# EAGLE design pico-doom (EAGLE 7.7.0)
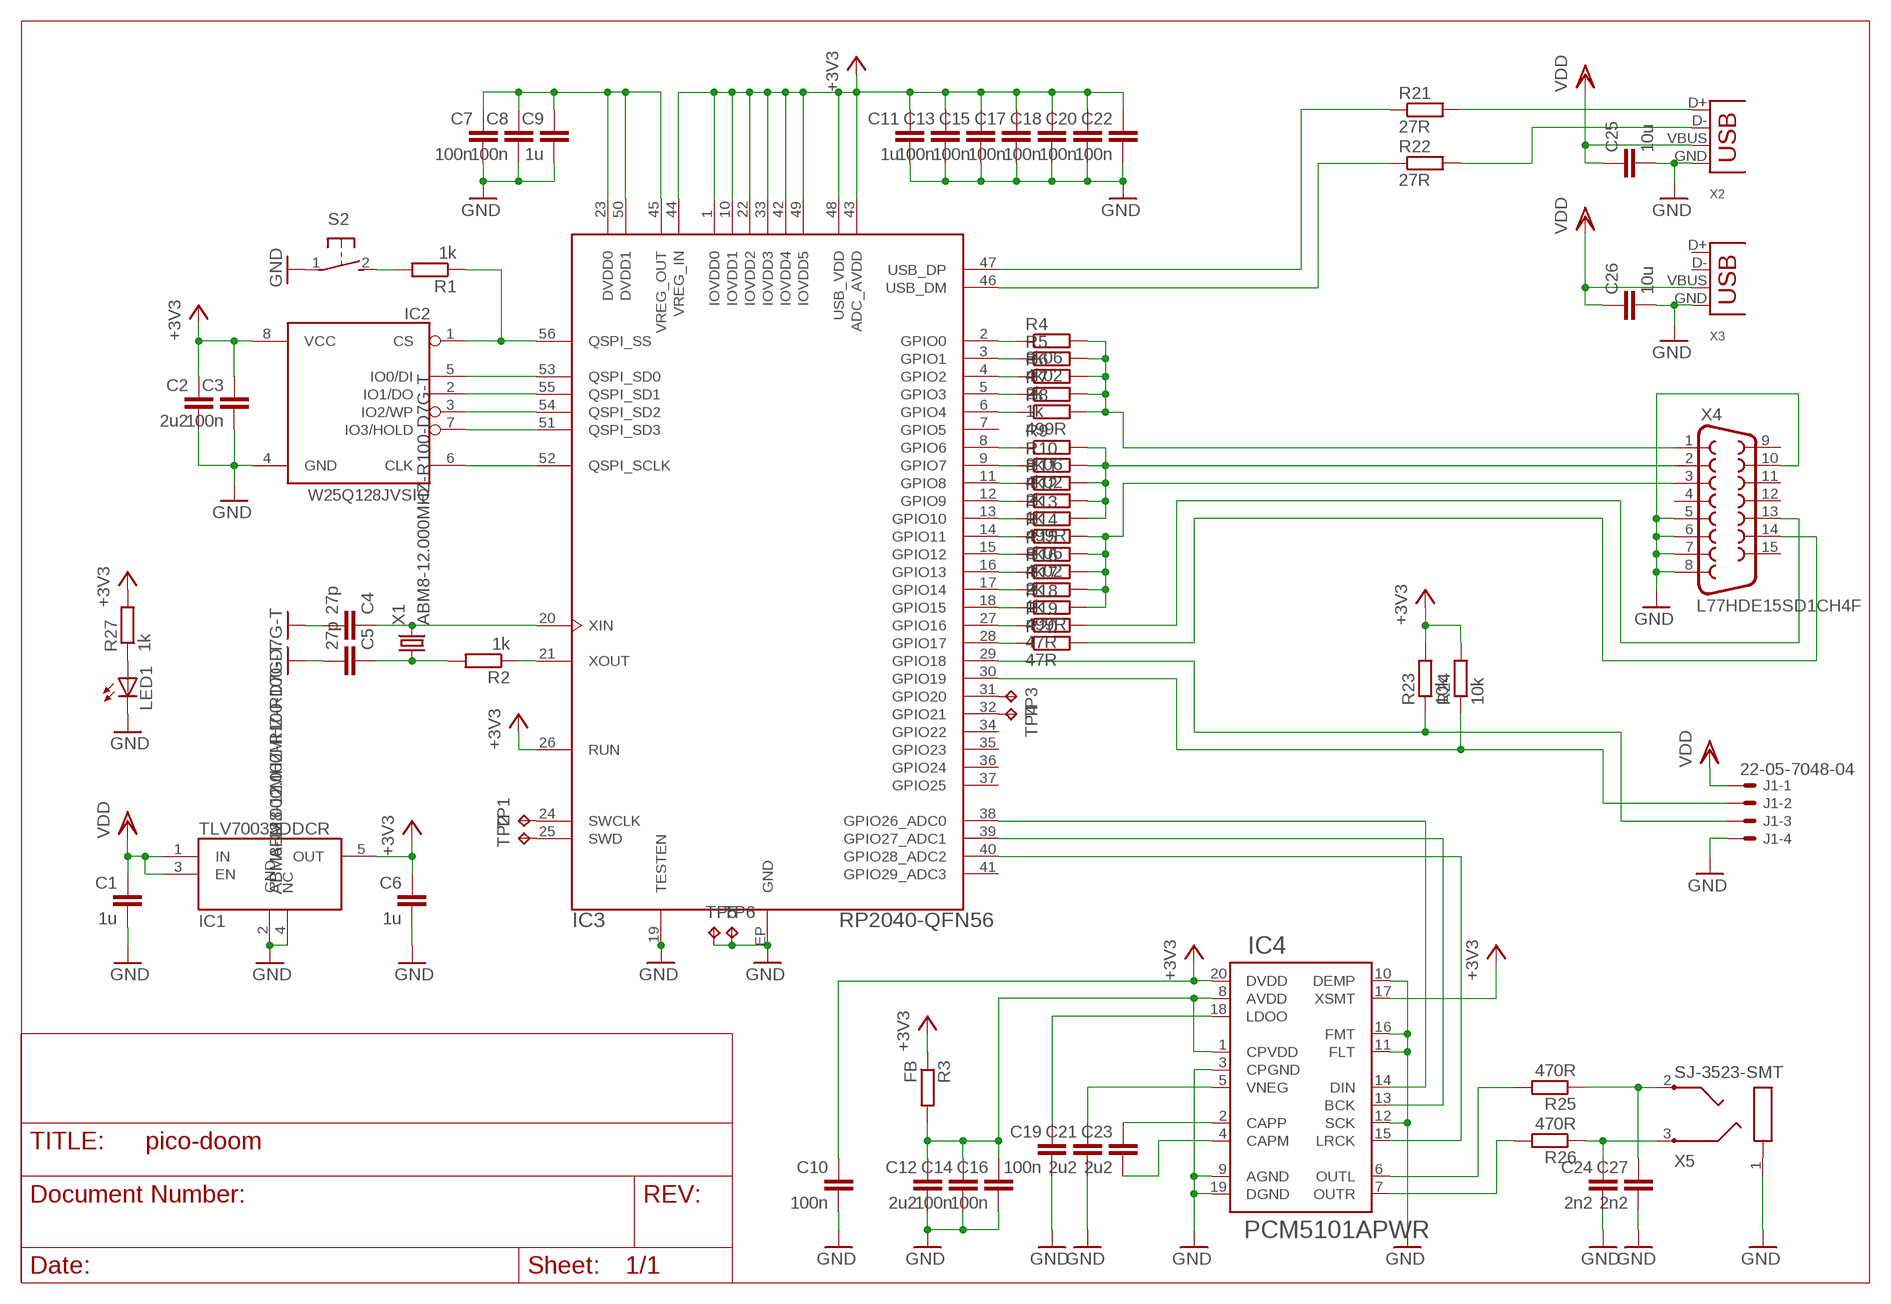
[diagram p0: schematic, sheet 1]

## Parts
C1  1u  C-EUC0603  [C0603]
C2  2u2  C-EUC0603  [C0603]
C3  100n  C-EUC0603  [C0603]
C4  27p  C-EUC0603  [C0603]
C5  27p  C-EUC0603  [C0603]
C6  1u  C-EUC0603  [C0603]
C7  100n  C-EUC0603  [C0603]
C8  100n  C-EUC0603  [C0603]
C9  1u  C-EUC0603  [C0603]
C10  100n  C-EUC0603  [C0603]
C11  1u  C-EUC0603  [C0603]
C12  2u2  C-EUC0603  [C0603]
C13  100n  C-EUC0603  [C0603]
C14  100n  C-EUC0603  [C0603]
C15  100n  C-EUC0603  [C0603]
C16  100n  C-EUC0603  [C0603]
C17  100n  C-EUC0603  [C0603]
C18  100n  C-EUC0603  [C0603]
C19  100n  C-EUC0603  [C0603]
C20  100n  C-EUC0603  [C0603]
C21  2u2  C-EUC0603  [C0603]
C22  100n  C-EUC0603  [C0603]
C23  2u2  C-EUC0603  [C0603]
C24  2n2  C-EUC0603  [C0603]
C25  10u  C-EUC0805K  [C0805K]
C26  10u  C-EUC0805K  [C0805K]
C27  2n2  C-EUC0603  [C0603]
IC1  TLV70033DDCR  [SOT23-5]
IC2  W25Q128JVSIQ  [SO-08M]
IC3  RP2040-QFN56  [RP2040-QFN-56]
IC4  PCM5101APWR  PCM5102A  [TSSOP-20]
J1  22-05-7048-04  [7395-04]
LED1  LEDCHIP-LED0603  [CHIP-LED0603]
R1  1k  R-EU_R0603  [R0603]
R2  1k  R-EU_R0603  [R0603]
R3  FB  R-EU_R0603  [R0603]
R4  8k06  R-EU_R0603  [R0603]
R5  4k02  R-EU_R0603  [R0603]
R6  2k  R-EU_R0603  [R0603]
R7  1k  R-EU_R0603  [R0603]
R8  499R  R-EU_R0603  [R0603]
R9  8k06  R-EU_R0603  [R0603]
R10  4k02  R-EU_R0603  [R0603]
R11  2k  R-EU_R0603  [R0603]
R12  1k  R-EU_R0603  [R0603]
R13  499R  R-EU_R0603  [R0603]
R14  8k06  R-EU_R0603  [R0603]
R15  4k02  R-EU_R0603  [R0603]
R16  2k  R-EU_R0603  [R0603]
R17  1k  R-EU_R0603  [R0603]
R18  499R  R-EU_R0603  [R0603]
R19  47R  R-EU_R0603  [R0603]
R20  47R  R-EU_R0603  [R0603]
R21  27R  R-EU_R0603  [R0603]
R22  27R  R-EU_R0603  [R0603]
R23  10k  R-EU_R0603  [R0603]
R24  10k  R-EU_R0603  [R0603]
R25  470R  R-EU_R0603  [R0603]
R26  470R  R-EU_R0603  [R0603]
R27  1k  R-EU_R0603  [R0603]
S2  PTS636-SM25F  [PTS636]
TP1  TPB1,27  [B1,27]
TP2  TPB1,27  [B1,27]
TP3  TPB1,27  [B1,27]
TP4  TPB1,27  [B1,27]
TP5  TPB1,27  [B1,27]
TP6  TPB1,27  [B1,27]
X1  ABM8-12.000MHZ-R100-D7G-T  XTAL-3225  [SMD3225]
X2  SS-52100-001  USB-A-H  [USB-A-H]
X3  MINI  USB-MB-S  [USB-MB-S]
X4  L77HDE15SD1CH4F  F15HDH  [HDF15H]
X5  SJ-3523-SMT  [SJ-3523-SMT]

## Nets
+3V3: C2.1 C3.1 C6.1 C10.1 C11.1 C13.1 C15.1 C17.1 C18.1 C20.1 C22.1 IC1.5(OUT) IC2.8(VCC) IC3.1(IOVDD0) IC3.10(IOVDD1) IC3.22(IOVDD2) IC3.26(RUN) IC3.33(IOVDD3) IC3.42(IOVDD4) IC3.43(ADC_AVDD) IC3.44(VREG_IN) IC3.48(USB_VDD) IC3.49(IOVDD5) IC4.17(XSMT) IC4.20(DVDD) R3.1 R23.2 R24.2 R27.2
AVDD: C12.1 C14.1 C16.1 IC4.1(CPVDD) IC4.8(AVDD) R3.2
DVDD: C7.1 C8.1 C9.1 IC3.23(DVDD0) IC3.45(VREG_OUT) IC3.50(DVDD1)
GND: C1.2 C2.2 C3.2 C4.2 C5.2 C6.2 C7.2 C8.2 C9.2 C10.2 C11.2 C12.2 C13.2 C14.2 C15.2 C16.2 C17.2 C18.2 C19.2 C20.2 C21.2 C22.2 C24.2 C25.2 C26.2 C27.2 IC1.2(GND) IC1.4(NC) IC2.4(GND) IC3.19(TESTEN) IC3.EP(GND) IC4.3(CPGND) IC4.9(AGND) IC4.10(DEMP) IC4.11(FLT) IC4.12(SCK) IC4.16(FMT) IC4.19(DGND) J1.4 LED1.C S2.1(P) TP5.TP TP6.TP X1.2(GND) X1.4(GND) X2.GND X3.GND X4.5 X4.6 X4.7 X4.8 X4.10 X5.1(S)
N$1: R4.2 R5.2 R6.2 R7.2 R8.2 X4.1
N$2: IC2.5(IO0/DI) IC3.53(QSPI_SD0)
N$3: IC2.2(IO1/DO) IC3.55(QSPI_SD1)
N$4: IC2.7(IO3/HOLD) IC3.51(QSPI_SD3)
N$5: IC2.3(IO2/WP) IC3.54(QSPI_SD2)
N$6: IC2.6(CLK) IC3.52(QSPI_SCLK)
N$7: R1.2 S2.2(S)
N$8: LED1.A R27.1
N$9: IC3.39(GPIO27_ADC1) IC4.13(BCK)
N$10: C4.1 IC3.20(XIN) X1.3
N$11: C5.1 R2.2 X1.1
N$12: IC3.21(XOUT) R2.1
N$13: IC3.27(GPIO16) R19.1
N$14: R19.2 X4.13
N$15: IC3.46(USB_DM) R22.1
N$16: IC3.47(USB_DP) R21.1
N$17: IC3.2(GPIO0) R4.1
N$18: IC3.3(GPIO1) R5.1
N$19: IC3.4(GPIO2) R6.1
N$20: IC3.5(GPIO3) R7.1
N$21: IC3.6(GPIO4) R8.1
N$22: IC3.24(SWCLK) TP1.TP
N$23: IC3.8(GPIO6) R9.1
N$24: IC3.9(GPIO7) R10.1
N$25: IC3.11(GPIO8) R11.1
N$26: IC3.12(GPIO9) R12.1
N$27: IC3.13(GPIO10) R13.1
N$28: R9.2 R10.2 R11.2 R12.2 R13.2 X4.2
N$29: IC3.14(GPIO11) R14.1
N$30: IC3.15(GPIO12) R15.1
N$31: IC3.16(GPIO13) R16.1
N$32: IC3.17(GPIO14) R17.1
N$33: IC3.18(GPIO15) R18.1
N$34: R14.2 R15.2 R16.2 R17.2 R18.2 X4.3
N$35: IC3.28(GPIO17) R20.1
N$36: R20.2 X4.14
N$37: IC4.6(OUTL) R25.2
N$39: C23.1 IC4.2(CAPP)
N$40: C23.2 IC4.4(CAPM)
N$41: C21.1 IC4.5(VNEG)
N$42: IC3.40(GPIO28_ADC2) IC4.15(LRCK)
N$43: IC4.7(OUTR) R26.2
N$44: C24.1 R26.1 X5.3(R)
N$45: C27.1 R25.1 X5.2(T)
N$46: IC3.38(GPIO26_ADC0) IC4.14(DIN)
N$48: C19.1 IC4.18(LDOO)
N$49: IC3.25(SWD) TP2.TP
N$52: R22.2 X2.D-
N$53: R21.2 X2.D+
N$55: IC3.29(GPIO18) J1.3 R23.1
N$56: IC3.30(GPIO19) J1.2 R24.1
N$57: IC2.1(CS) IC3.56(QSPI_SS) R1.1
N$58: IC3.31(GPIO20) TP3.TP
N$59: IC3.32(GPIO21) TP4.TP
VDD: C1.1 C25.1 C26.1 IC1.1(IN) IC1.3(EN) J1.1 X2.VBUS X3.VBUS
Unconnected: IC3.7(GPIO5) IC3.34(GPIO22) IC3.35(GPIO23) IC3.36(GPIO24) IC3.37(GPIO25) IC3.41(GPIO29_ADC3) X3.D+ X3.D- X4.4 X4.9 X4.11 X4.12 X4.15

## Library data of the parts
C1-C27 = rcl:C-EU: CAPACITOR, European symbol
IC1 = pico-doom:TLV70033DDCR
IC2 = pico-doom:W25Q128JVSIQ
IC3 = pico-doom:RP2040-QFN56
IC4 = pico-doom:PCM5102A
J1 = con-molex:22-?-04: CONNECTOR wire to board 2.54 mm (.1 inch) pitch header; OC_FARNELL: unknown; OC_NEWARK: unknown
LED1 = led:LED: LED
R1-R27 = rcl:R-EU_: RESISTOR, European symbol
S2 = pico-doom:PTS636: OMRON SWITCH
TP1-TP6 = testpad:TP: Test pad
X1 = pico-doom:XTAL-3225
X2 X3 = con-usb-3:USB: USB Connectors
X4 = con-subd:F15: SUB-D; OC_FARNELL: unknown; OC_NEWARK: unknown
X5 = pico-doom:SJ-3523-SMT: MIC/HEADPHONE JACK KS-S stereo microphone/headphone jack PG203JN (Schukat)

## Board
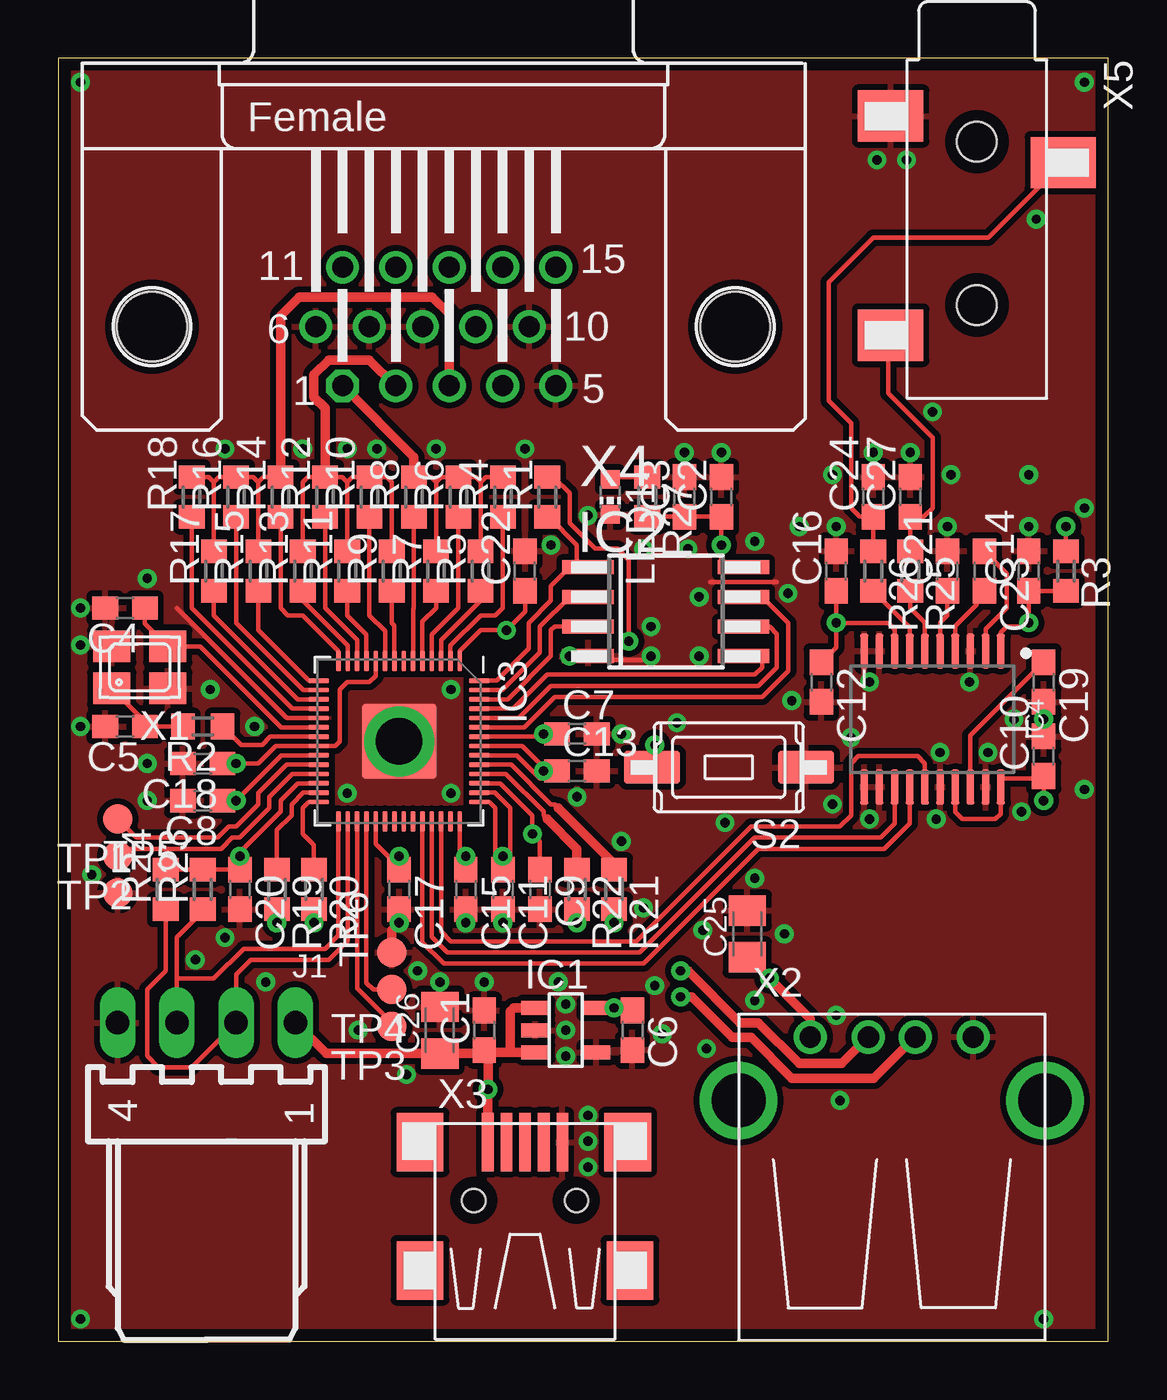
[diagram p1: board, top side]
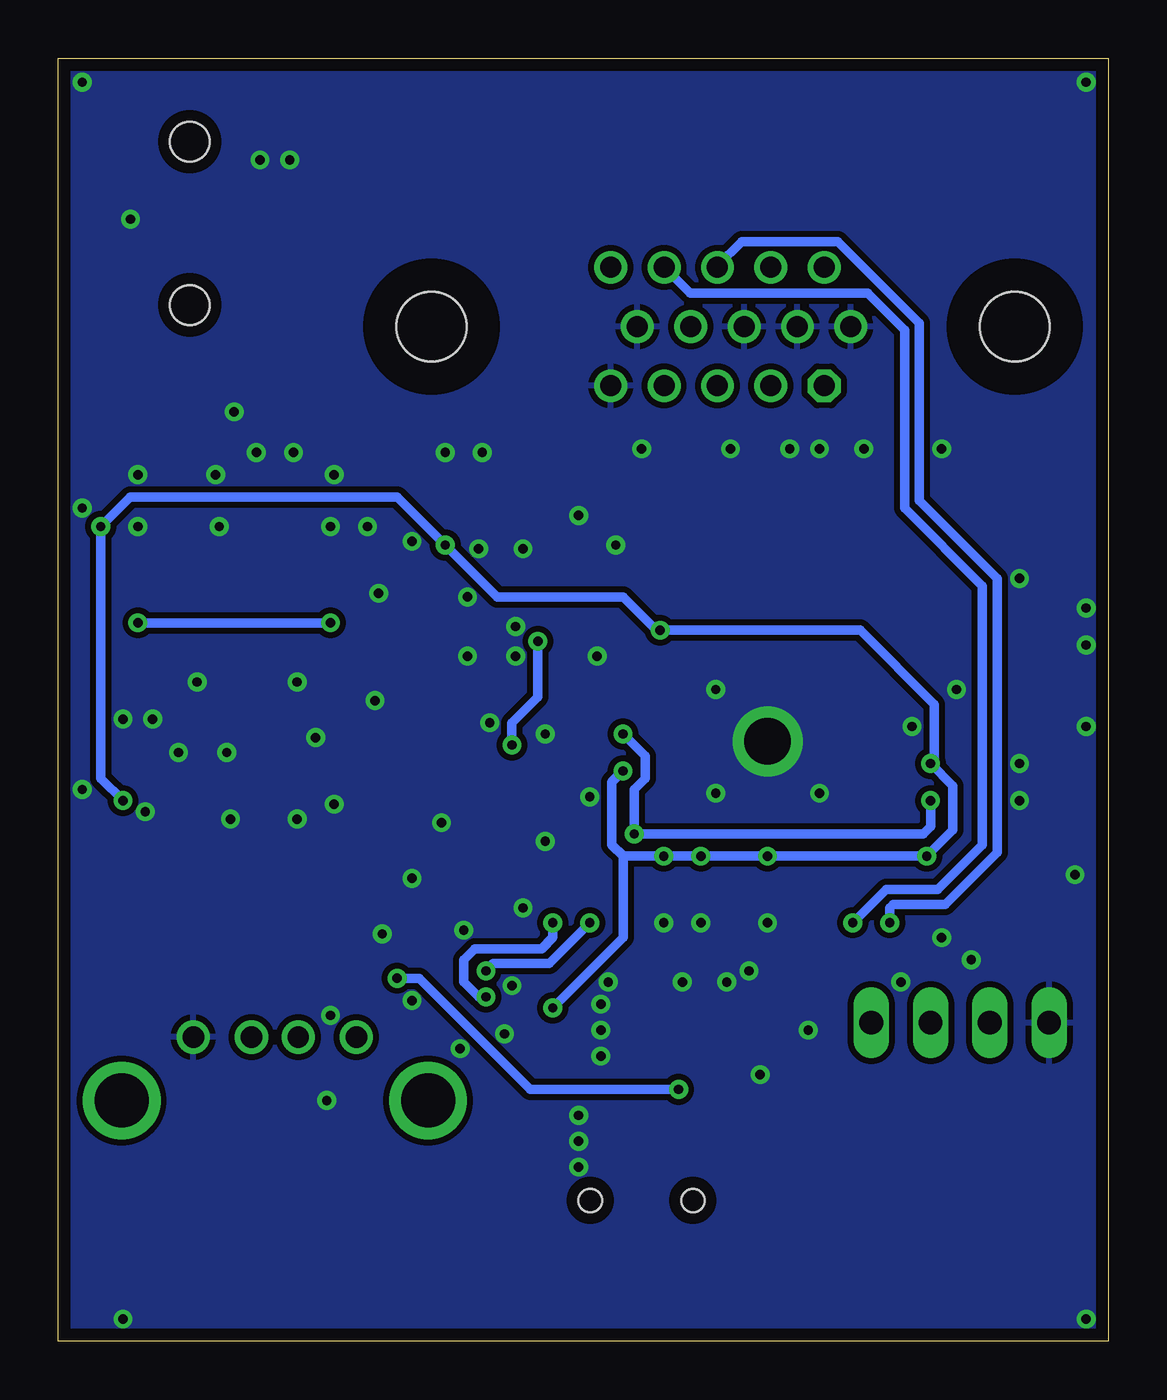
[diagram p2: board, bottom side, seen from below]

Size 45 x 55 mm. Coordinates in mm from the lower left corner, seen from the top.
Outline: 0,0 45,0 45,55 0,55 0,0
Copper layers (1*16): Top 0.035mm / dielectric 1.5mm / Bottom 0.035mm
Design rules "default *": minimum track width 0.2mm, minimum drill 0.4mm, track to track 0.2mm, track to pad 0.2mm, pad to pad 0.2mm, via to via 0.2mm, smd to smd 0mil, copper to edge 20mil, drill to drill 0.2mm, minimum pad ring 10mil, minimum via ring 8mil, stop-mask expansion 0.05mm, vias tented up to drill 0.4mm, thermal gap 10mil

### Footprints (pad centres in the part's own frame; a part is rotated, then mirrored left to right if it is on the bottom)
C0603 = smd 1.1 x 1: 1 -0.85,0; 2 0.85,0
C0805K = smd 1.3 x 1.6: 1 -1,0; 2 1,0
SOT23-5 = smd 0.6 x 1.2: 1 -0.95,-1.306; 2 0,-1.306; 3 0.95,-1.306; 4 0.95,1.306; 5 -0.95,1.306
SO-08M = smd 0.6 x 2.2: 1 -1.905,-3.33; 2 -0.635,-3.33; 3 0.635,-3.33; 4 1.905,-3.33; 5 1.905,3.33; 6 0.635,3.33; 7 -0.635,3.33; 8 -1.905,3.33
RP2040-QFN-56 = smd 0.875 x 0.2: 1 -3.438,2.6; 2 -3.438,2.2; 3 -3.438,1.8; 4 -3.438,1.4; 5 -3.438,1; 6 -3.438,0.6; 7 -3.438,0.2; 8 -3.438,-0.2; 9 -3.438,-0.6; 10 -3.438,-1; 11 -3.438,-1.4; 12 -3.438,-1.8; 13 -3.438,-2.2; 14 -3.438,-2.6; 29 3.438,-2.6; 30 3.438,-2.2; 31 3.438,-1.8; 32 3.438,-1.4; 33 3.438,-1; 34 3.438,-0.6; 35 3.438,-0.2; 36 3.438,0.2; 37 3.438,0.6; 38 3.438,1; 39 3.438,1.4; 40 3.438,1.8; 41 3.438,2.2; 42 3.438,2.6 | smd 0.2 x 0.875: 15 -2.6,-3.438; 16 -2.2,-3.438; 17 -1.8,-3.438; 18 -1.4,-3.438; 19 -1,-3.438; 20 -0.6,-3.438; 21 -0.2,-3.438; 22 0.2,-3.438; 23 0.6,-3.438; 24 1,-3.438; 25 1.4,-3.438; 26 1.8,-3.438; 27 2.2,-3.438; 28 2.6,-3.438; 43 2.6,3.438; 44 2.2,3.438; 45 1.8,3.438; 46 1.4,3.438; 47 1,3.438; 48 0.6,3.438; 49 0.2,3.438; 50 -0.2,3.438; 51 -0.6,3.438; 52 -1,3.438; 53 -1.4,3.438; 54 -1.8,3.438; 55 -2.2,3.438; 56 -2.6,3.438 | smd 3.2 x 3.2: EP 0,0
TSSOP-20 = smd 1.5 x 0.35: 1 -2.918,2.925; 2 -2.918,2.275; 3 -2.918,1.625; 4 -2.918,0.975; 5 -2.918,0.325; 6 -2.918,-0.325; 7 -2.918,-0.975; 8 -2.918,-1.625; 9 -2.918,-2.275; 10 -2.918,-2.925; 11 2.918,-2.925; 12 2.918,-2.275; 13 2.918,-1.625; 14 2.918,-0.975; 15 2.918,-0.325; 16 2.918,0.325; 17 2.918,0.975; 18 2.918,1.625; 19 2.918,2.275; 20 2.918,2.925
7395-04 = drill 1.016 long: 1 3.81,0; 2 1.27,0; 3 -1.27,0; 4 -3.81,0
CHIP-LED0603 = smd 0.8 x 0.8: A 0,-0.75; C 0,0.75
R0603 = smd 1 x 1.1: 1 -0.85,0; 2 0.85,0
PTS636 = smd 2.4 x 1.4: 1 -3.3,0; 2 3.3,0
B1,27 = smd 1.27 x 1.27: TP 0,0
SMD3225 = smd 1.6 x 1.35: 1 1.2,0.9; 2 -1.2,0.9; 3 -1.2,-0.9; 4 1.2,-0.9
USB-A-H = drill 0.914: D+ 2.718,-1.003; D- 2.718,1.003; GND 2.718,-3.493; VBUS 2.718,3.493 | drill 2.311: P$5 0,-6.566; P$6 0,6.566
USB-MB-S = smd 2.5 x 0.5: D+ 2.5,0; D- 2.5,0.8; GND 2.5,-1.6; ID 2.5,-0.8; VBUS 2.5,1.6 | smd 2.5 x 2: P$1 -3,-4.5; P$2 -3,4.5; P$3 2.5,-4.4; P$4 2.5,4.5 | hole 1: 0,2.2; 0,-2.2
HDF15H = drill 0.9 octagon: 1 4.329,2.54 | drill 0.9: 2 2.043,2.54; 3 -0.243,2.54; 4 -2.529,2.54; 5 -4.815,2.54; 6 5.472,0; 7 3.186,0; 8 0.9,0; 9 -1.386,0; 10 -3.672,0; 11 4.329,-2.54; 12 2.043,-2.54; 13 -0.243,-2.54; 14 -2.529,-2.54; 15 -4.815,-2.54 | hole 3: -12.5,0; 12.5,0
SJ-3523-SMT = smd 2.2 x 2.8: 1 2.4,-3.7; 2 11.8,-3.7; 3 4.4,3.7 | hole 1.7: 3.5,0; 10.5,0

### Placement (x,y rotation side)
C1  18.26,13.34 90 top
C2  28.42,36.2 90 top
C3  26.83,36.2 90 top
C4  2.86,31.43 180 top
C5  2.86,26.35 180 top
C6  24.61,13.34 270 top
C7  22.23,26.04 0 top
C8  6.19,23.18 180 top
C9  20.64,19.37 270 top
C10  42.23,25.08 90 top
C11  19.05,19.37 270 top
C12  32.7,28.26 270 top
C13  22.23,24.45 0 top
C14  41.59,33.02 90 top
C15  17.46,19.37 270 top
C16  33.34,33.02 90 top
C17  14.61,19.37 270 top
C18  6.19,24.77 180 top
C19  42.23,28.26 270 top
C20  7.78,19.37 270 top
C21  38.1,33.02 90 top
C22  20,33.02 90 top
C23  39.69,33.02 270 top
C24  34.92,36.2 90 top
C25  29.53,17.46 90 top
C26  16.35,13.34 90 top
C27  36.51,36.2 90 top
IC1  21.75,13.34 270 top
IC2  26.04,31.27 270 top
IC3  14.61,25.72 270 top
IC4  37.47,26.67 270 top
J1  6.35,13.65 0 top
LED1  23.65,36.2 180 top
R1  20.95,36.2 90 top
R2  6.19,26.35 180 top
R3  43.18,33.02 270 top
R4  19.05,36.2 90 top
R5  18.1,33.02 90 top
R6  17.14,36.2 90 top
R7  16.19,33.02 90 top
R8  15.24,36.2 90 top
R9  14.29,33.02 90 top
R10  13.34,36.2 90 top
R11  12.38,33.02 90 top
R12  11.43,36.2 90 top
R13  10.48,33.02 90 top
R14  9.53,36.2 90 top
R15  8.57,33.02 90 top
R16  7.62,36.2 90 top
R17  6.67,33.02 90 top
R18  5.71,36.2 90 top
R19  9.37,19.37 270 top
R20  10.95,19.37 270 top
R21  23.81,19.37 270 top
R22  22.23,19.37 270 top
R23  6.19,19.37 90 top
R24  4.6,19.37 90 top
R25  36.51,33.02 270 top
R26  34.92,33.02 270 top
R27  25.24,36.2 270 top
S2  28.73,24.61 180 top
TP1  2.54,22.38 180 top
TP2  2.54,20.8 180 top
TP3  14.29,13.49 180 top
TP4  14.29,15.08 180 top
TP5  2.54,19.21 0 top
TP6  14.29,16.67 90 top
X1  3.49,28.89 180 top
X2  35.72,10.32 90 top
X3  20,6.03 90 top
X4  16.51,43.5 180 top
X5  39.37,54.93 270 top

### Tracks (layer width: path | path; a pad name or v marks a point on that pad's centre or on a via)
+3V3  (via drill 0.4)
  Top 0.2: IC3.10 13.61,28.53 13.34,28.26 12.38,28.26 12.06,27.94 12.06,25.72 11.87,25.52 IC3.22 9.32,25.52 8.57,24.77 v7.62,24.77 C18.1 | IC3.42 17.2,20.64 | 17.2,20.64 17.2,20.48 C15.1 | C11.1 19.05,20.32 18.73,20.64 18.73,22.86 18.48,23.12 IC3.43 | IC3.44 18.71,23.52 19.37,22.86 19.37,20.54 C11.1 | IC3.48 19.65,25.12 20.64,24.13 21.06,24.13 C13.1 | IC3.49 19.89,25.52 20.64,24.77 21.06,24.77 C13.1 | IC3.33 13.61,21.32 14.61,20.32 | C17.1 14.61,20.32 | IC3.26 10.27,23.92 9.53,23.18 9.53,22.7 7.78,20.95 v7.78,20.8 C20.1 R23.2 R24.2 | IC3.1 17.2,29.59 18.1,30.48 v19.21,30.48 20,31.27 C22.1 | v19.05,20.8 C11.1 | v17.46,20.8 17.36,20.8 17.2,20.64 | v20.8,24.45 C13.1 | 14.61,20.32 v14.61,20.8 | IC4.17 38.44,22.68 38.73,22.38 40.16,22.38 40.39,22.61 IC4.20 40.39,24.06 40.32,24.13 42.12,24.13 C10.1 v42.23,23.18 | R3.1 v43.18,34.92 | R27.2 C3.1 | C3.1 26.83,35.24 | C2.1 28.42,35.24 | C3.1 C2.1 | C2.1 v28.42,34.13 28.42,33.18 IC2.8
  Top 0.406: IC1.5 24.51,14.29 C6.1 24.5,14.29 v23.81,14.29
  Bottom 0.406: v20.8,24.45 21.27,23.97 21.27,21.27 20.8,20.8 | 20.8,20.8 v19.05,20.8 v17.46,20.8 v14.61,20.8 v7.78,20.8 6.67,21.91 6.67,23.81 v7.62,24.77 7.46,24.92 7.46,27.3 10.64,30.48 v19.21,30.48 19.37,30.48 20.8,31.91 26.19,31.91 v28.42,34.13 30.48,36.2 41.91,36.2 v43.18,34.92 43.18,24.13 v42.23,23.18 | v23.81,14.29 20.8,17.3 20.8,20.8
AVDD  (via drill 0.4)
  Top 0.2: IC4.1 40.39,30.39 40.64,30.64 41.59,30.64 v41.59,30.8 C14.1 R3.2 | IC4.8 35.84,30.52 35.56,30.8 v33.34,30.8 | C12.1 33.34,29.74 v33.34,30.8 | C16.1 v33.34,30.8
  Bottom 0.406: v33.34,30.8 v41.59,30.8
DVDD  (via drill 0.4)
  Top 0.2: IC3.45 18.95,23.92 20.32,22.54 v20.32,21.75 20.64,21.43 C9.1 | IC3.23 9.56,25.12 v7.62,23.18 C8.1 | IC3.50 20.68,25.92 v20.8,26.04 C7.1
  Bottom 0.406: v20.8,26.04 19.84,25.08 19.84,24.13 20.32,23.65 v20.32,21.75 7.94,21.75 7.62,22.07 v7.62,23.18
GND  (via drill 0.4, 2)
  Top 0.2: IC3.19 9.79,26.72 5.08,31.43 | v25.4,29.37 25.24,29.21 22.86,29.21 IC2.4 | 27.94,32.54 30.8,32.54
  Top 0.406: TP6.TP 14.29,17.62 v14.61,17.94
  other vias: 34.77,22.38 37.78,25.24 37.62,22.38 43.97,23.65 39.05,28.26 34.77,28.26 34.92,38.1 36.51,38.1 31.75,34.92 41.59,34.92 38.1,34.92 33.34,34.92 14.61,25.72 7.14,17.3 26.83,38.1 21.11,34.13 16.19,38.26 10.48,38.26 7.14,38.26 6.51,27.94 0.95,26.35 0.95,31.43 3.81,24.77 3.81,23.18 12.38,23.5 16.83,23.5 16.83,27.94 16.35,15.4 8.89,15.4 22.7,8.57 22.7,7.46 22.7,9.68 27.78,12.54 29.84,14.61 28.57,22.23 29.84,19.84 25.88,13.18 25.08,18.57 24.13,26.04 18.26,15.4 21.75,13.34 21.75,14.45 21.75,12.22 33.18,23.02 33.97,25.88 33.5,10.32 14.92,11.43 22.23,23.34 43.97,53.98 41.91,48.1 37.47,39.85 35.08,50.64 36.35,50.64 12.38,38.26 13.65,38.26 5.87,16.35 19.05,17.94 17.46,17.94 20,38.26 40.96,26.67 1.43,20 15.4,15.88 12.86,13.34 27.62,17.62 33.34,13.97 25.56,15.24 21.43,15.4 24.13,21.43 3.81,32.7 0.95,29.84 31.27,32.07 29.84,34.29 8.41,26.35 26.51,26.51 39.85,25.24 42.23,26.67 38.26,37.15 41.59,37.15 33.18,37.15 31.43,27.46 28.42,38.1 43.97,35.72 41.27,22.7 31.11,17.46 22.7,35.4 25.4,30.64 25.08,33.97 21.91,29.37 0.95,0.95 42.23,0.95 0.95,53.98 26.99,33.97 27.46,29.37 27.46,31.91
  pour Top (isolate 0.254): 0,0 45.09,0 45.09,54.93 0,54.93
  pour Bottom (isolate 0.254): 0,0 45.09,0 45.09,54.93 0,54.93
  pour Top (isolate 0.254, rank 2, no thermals): 12.7,27.62 16.51,27.62 16.51,23.81 12.7,23.81
N$1
  Top 0.2: R5.2 18.1,36.83 | R7.2 16.19,36.83 | R4.2 18.31,37.05 18.1,36.83 | 18.1,36.83 17.88,37.05 R6.2 16.41,37.05 16.19,36.83 | R8.2 15.98,37.05 16.19,36.83
  Top 0.406: R8.2 15.24,37.9 X4.1
N$2
  Top 0.2: IC3.53 19.5,27.12 20.95,28.57 29.84,28.57 30.16,28.89 30.16,29.37 IC2.5
N$3
  Top 0.2: IC2.2 21.91,31.91 20.64,30.64 20.64,29.53 19.03,27.92 IC3.55
N$4
  Top 0.2: IC3.51 19.97,26.32 21.27,27.62 30.16,27.62 31.27,28.73 31.27,30.8 30.16,31.91 IC2.7
N$5
  Top 0.2: IC3.54 19.26,27.52 21.11,29.37 21.11,30.48 21.27,30.64 IC2.3
N$6
  Top 0.2: IC3.52 19.73,26.72 21.11,28.1 30,28.1 30.8,28.89 30.8,30.32 30.48,30.64 IC2.6
N$7  (via drill 0.4)
  Top 0.2: R1.2 21.22,37.05 21.91,36.35 21.91,35.08 23.02,33.97 23.97,33.97 24.45,33.5 v24.45,30 | v25.56,25.56 25.56,24.73 S2.2
  Bottom 0.406: v24.45,30 24.45,27.62 25.56,26.51 v25.56,25.56
N$8
  Top 0.2: R27.1 23.75,37.05 LED1.A
N$9
  Top 0.2: IC3.39 16,17.33 16.67,16.67 24.92,16.67 29.84,21.59 35.24,21.59 35.84,22.19 IC4.13
N$10
  Top 0.2: IC3.20 9.56,26.32 6.08,29.79 X1.3 3.71,30.78 C4.1
N$11
  Top 0.2: R2.2 C5.1 3.71,26.58 X1.1
N$12
  Top 0.2: IC3.21 9.09,25.92 8.73,25.56 7.83,25.56 R2.1
N$13
  Top 0.2: IC3.27 10.5,23.52 10,23.02 10,22.54 9.37,21.91 R19.1
N$14  (via drill 0.4)
  Top 0.406: R19.2 v9.37,17.94
  Bottom 0.2: X4.13 16.75,46.11
  Bottom 0.406: 16.75,46.11 15.72,47.15 11.59,47.15 8.1,43.66 8.1,36.04 4.76,32.7 4.76,20.95 6.99,18.73 9.21,18.73 9.37,18.57 v9.37,17.94
N$15
  Top 0.2: IC3.46 19.18,24.32 20.8,22.7 20.8,22.54 20.95,22.38
  Top 0.406: R22.1 22.23,21.11 20.95,22.38
N$16
  Top 0.2: IC3.47 19.41,24.72 21.11,23.02 21.27,23.02 21.43,22.86
  Top 0.406: R21.1 23.81,20.48 21.43,22.86
N$17
  Top 0.2: IC3.2 16.8,29.82 18.1,31.11 18.73,31.11 19.05,31.43 R4.1
N$18
  Top 0.2: IC3.3 16.41,30.06 18.1,31.75 R5.1 18.1,32.07
N$19
  Top 0.2: IC3.4 16,30.29 17.14,31.43 R6.1
N$20
  Top 0.2: 16.19,31.75 R7.1 16.19,31.43 15.61,30.84 IC3.5
N$21
  Top 0.2: R8.1 15.24,31.43 15.21,31.4 IC3.6
N$22
  Top 0.2: IC3.24 9.79,24.72 8.57,23.5 8.57,23.02 7.62,22.07 7.3,22.07 6.83,21.59 3.33,21.59 TP1.TP
N$23
  Top 0.2: 14.09,31.97 R9.1 14.29,30.8 14.4,30.68 IC3.8
N$24
  Top 0.2: IC3.9 14.01,30.45 13.34,31.11 R10.1
N$25
  Top 0.2: IC3.11 13.21,30.29 12.38,31.11 R11.1
N$26
  Top 0.2: IC3.12 12.8,30.06 11.43,31.43 R12.1
N$27
  Top 0.2: IC3.13 12.4,29.82 10.48,31.75 R13.1
N$28
  Top 0.2: R9.2 14.29,36.83 14.07,37.05 R10.2 12.6,37.05 12.38,36.83 | R11.2 12.38,36.83 | R13.2 10.48,36.83 10.69,37.05 R12.2 12.17,37.05 12.38,36.83
  Top 0.406: X4.2 14.45,40.96 13.34,42.07 11.59,42.07 10.95,41.43 10.95,40.48 11.43,40.01 R12.2
N$29
  Top 0.2: IC3.14 12.01,29.59 10.48,31.11 9.84,31.11 9.53,31.43 R14.1
N$30
  Top 0.2: IC3.15 10.73,28.32 8.57,30.48 R15.1 8.52,32.17
N$31
  Top 0.2: IC3.16 10.5,27.92 7.62,30.8 R16.1
N$32
  Top 0.2: IC3.17 10.27,27.52 6.67,31.11 R17.1
N$33
  Top 0.2: IC3.18 10.03,27.12 5.71,31.43 R18.1
N$34
  Top 0.2: R15.2 8.57,36.83 | R17.2 6.67,36.83 | R14.2 8.79,37.05 8.57,36.83 | 8.57,36.83 8.36,37.05 R16.2 6.88,37.05 6.67,36.83 | R18.2 6.45,37.05 6.67,36.83
  Top 0.406: X4.3 16.75,44.05 16.03,44.77 10.32,44.77 9.53,43.97 R14.2
N$35
  Top 0.2: IC3.28 10.73,23.12 10.48,22.86 10.48,21.75 10.95,21.27 R20.1
N$36  (via drill 0.4)
  Top 0.406: R20.2 v10.95,17.94
  Bottom 0.406: X4.14 17.93,44.93 10.32,44.93 8.73,43.34 8.73,35.72 5.4,32.38 5.4,21.27 7.3,19.37 9.53,19.37 v10.95,17.94
N$37
  Top 0.2: IC4.6 37.14,30.8 36.51,31.43 R25.2
N$39
  Top 0.2: IC4.2 39.74,30.53 40.64,31.43 40.64,32.92 C23.1
N$40
  Top 0.2: IC4.4 38.44,30.66 39.37,31.59 39.37,31.85 C23.2
N$41
  Top 0.2: 38.1,31.75 C21.1 38.1,31.11 37.79,30.8 IC4.5
N$42
  Top 0.2: IC3.40 16.41,17.57 16.83,17.14 24.77,17.14 29.69,22.07 33.5,22.07 33.97,22.54 33.97,24.77 34.29,25.08 36.83,25.08 37.14,24.77 IC4.15
N$43
  Top 0.2: IC4.7 36.49,30.61 R26.2
N$44
  Top 0.2: X5.3 39.85,47.31 34.92,47.31 33.02,45.4 33.02,40.32 33.97,39.37 33.97,35.72 34.35,35.34 C24.1 R26.1
N$45
  Top 0.2: R25.1 C27.1 37.09,35.34 37.47,35.72 37.47,38.73 35.56,40.64 35.56,43.02
  Top 0.406: 35.56,43.02 X5.2
N$46
  Top 0.2: IC3.38 15.61,17.1 16.51,16.19 25.08,16.19 30,21.11 35.4,21.11 36.49,22.2 IC4.14
N$48
  Top 0.2: IC4.18 39.09,25.97 C19.1
N$49
  Top 0.2: IC3.25 10.03,24.32 9.05,23.34 9.05,22.86 7.78,21.59 7.46,21.59 6.99,21.11 2.86,21.11 TP2.TP 2.7,20.8
N$52  (via drill 0.4)
  Top 0.406: X2.D- 33.59,11.91 31.75,11.91 30,13.65 29.21,13.65 26.99,15.88 v26.67,15.88 | v22.23,17.94 R22.2
  Bottom 0.406: v26.67,15.88 26.35,16.19 23.97,16.19 v22.23,17.94
N$53  (via drill 0.4)
  Top 0.406: X2.D+ 34.96,11.27 31.43,11.27 29.69,13.02 28.89,13.02 27.15,14.76 v26.67,14.76 | v23.81,17.94 R21.2
  Bottom 0.406: v26.67,14.76 26.99,14.76 27.62,15.4 27.62,16.35 27.15,16.83 24.29,16.83 23.81,17.3 v23.81,17.94
N$55
  Top 0.2: IC3.29 12.01,17.4 11.43,16.83 7.94,16.83 6.67,15.56 5.08,15.56 | 5.08,15.56 5.08,17.3 6.19,18.41 R23.1 | 5.08,15.56 J1.3
N$56
  Top 0.2: IC3.30 12.4,17.17 11.59,16.35 8.26,16.35 7.62,15.72 J1.2 5.71,11.75 4.29,11.75 3.81,12.22 3.81,15.08 4.6,15.88 R24.1
N$57
  Top 0.2: 22.23,33.18 21.91,33.18 21.11,32.38 21.11,31.75 20.16,30.8 20.16,29.69 18.79,28.32 IC3.56 | 22.23,33.18 IC2.1 | R1.1 21.01,35.34 22.23,34.13 22.23,33.18
N$58
  Top 0.2: 14.23,13.44 TP3.TP 14.29,13.65 12.8,15.13 IC3.31
N$59
  Top 0.2: IC3.32 13.21,15.37 13.49,15.08 TP4.TP
VDD  (via drill 0.4)
  Top 0.406: J1.1 11.48,12.34 C26.1 18.11,12.34 C1.1 | IC1.3 19.37,12.38 | 19.37,12.38 18.36,12.38 C1.1 | IC1.1 19.52,14.29 19.37,14.13 19.37,12.38 | X3.VBUS v18.4,10.78 v18.41,10.79 18.41,12.33 C1.1 | X2.VBUS 32.23,13.81 v30.48,15.56 29.57,16.46 C25.1
  Bottom 0.406: v18.41,10.79 24.77,10.79 29.53,15.56 v30.48,15.56

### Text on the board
potisk: VGA | OK2ALP | AUDIO | 2023 | BOOT | RP2040 | I2C | POWER | KEYBRD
